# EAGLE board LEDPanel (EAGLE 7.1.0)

Size 152.65 x 130.18 mm. Coordinates in mm from the lower left corner, seen from the top.
Outline: 993 segments
Copper layers (1*16): Top 0.035mm / dielectric 1.5mm / Bottom 0.035mm
Design rules "default": minimum track width 10mil, minimum drill 24mil, track to track 8mil, track to pad 8mil, pad to pad 8mil, via to via 8mil, smd to smd 8mil, copper to edge 40mil, drill to drill 8mil, minimum pad ring 10mil, minimum via ring 8mil, stop-mask expansion 4mil, vias tented up to drill 0mil, thermal gap 10mil

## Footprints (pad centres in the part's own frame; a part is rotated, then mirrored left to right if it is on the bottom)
LED5MM = drill 0.813 octagon: A -1.27,0; K 1.27,0
SO14 = smd 0.6 x 2.2: 1 -3.81,-2.6; 2 -2.54,-2.6; 3 -1.27,-2.6; 4 0,-2.6; 5 1.27,-2.6; 6 2.54,-2.6; 7 3.81,-2.6; 8 3.81,2.6; 9 2.54,2.6; 10 1.27,2.6; 11 0,2.6; 12 -1.27,2.6; 13 -2.54,2.6; 14 -3.81,2.6
SA56-11 = drill 0.8 long: 1 -5.08,-7.62; 2 -2.54,-7.62; 3 0,-7.62; 4 2.54,-7.62; 5 5.08,-7.62; 6 5.08,7.62; 7 2.54,7.62; 8 0,7.62; 9 -2.54,7.62; 10 -5.08,7.62

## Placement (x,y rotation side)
E$1  [LED5MM]  124.84,73.03 90 top
E$2  [LED5MM]  132.46,73.03 90 top
E$3  [LED5MM]  109.6,73.03 90 top
E$4  [LED5MM]  117.22,73.03 90 top
E$5  [LED5MM]  94.36,73.03 90 top
E$6  [LED5MM]  101.98,73.03 90 top
E$7  [LED5MM]  79.12,73.03 90 top
E$8  [LED5MM]  86.74,73.03 90 top
E$9  [LED5MM]  63.88,73.03 90 top
E$10  [LED5MM]  71.5,73.03 90 top
E$11  [LED5MM]  48.64,73.03 90 top
E$12  [LED5MM]  56.26,73.03 90 top
E$13  [LED5MM]  33.4,73.03 90 top
E$14  [LED5MM]  41.02,73.03 90 top
E$15  [LED5MM]  18.16,73.03 90 top
E$16  [LED5MM]  25.78,73.03 90 top
E$17  [LED5MM]  124.84,80.64 90 top
E$18  [LED5MM]  132.46,80.64 90 top
E$19  [LED5MM]  109.6,80.64 90 top
E$20  [LED5MM]  117.22,80.64 90 top
E$21  [LED5MM]  94.36,80.64 90 top
E$22  [LED5MM]  101.98,80.64 90 top
E$23  [LED5MM]  79.12,80.64 90 top
E$24  [LED5MM]  86.74,80.64 90 top
E$25  [LED5MM]  63.88,80.64 90 top
E$26  [LED5MM]  71.5,80.64 90 top
E$27  [LED5MM]  48.64,80.64 90 top
E$28  [LED5MM]  56.26,80.64 90 top
E$29  [LED5MM]  33.4,80.64 90 top
E$30  [LED5MM]  41.02,80.64 90 top
E$31  [LED5MM]  18.16,80.64 90 top
E$32  [LED5MM]  25.78,80.64 90 top
E$33  [LED5MM]  124.84,88.27 90 top
E$34  [LED5MM]  132.46,88.27 90 top
E$35  [LED5MM]  109.6,88.27 90 top
E$36  [LED5MM]  117.22,88.27 90 top
E$37  [LED5MM]  94.36,88.27 90 top
E$38  [LED5MM]  101.98,88.27 90 top
E$39  [LED5MM]  79.12,88.27 90 top
E$40  [LED5MM]  86.74,88.27 90 top
E$41  [LED5MM]  63.88,88.27 90 top
E$42  [LED5MM]  71.5,88.27 90 top
E$43  [LED5MM]  48.64,88.27 90 top
E$44  [LED5MM]  56.26,88.27 90 top
E$45  [LED5MM]  33.4,88.27 90 top
E$46  [LED5MM]  41.02,88.27 90 top
E$47  [LED5MM]  18.16,88.27 90 top
E$48  [LED5MM]  25.78,88.27 90 top
E$49  [LED5MM]  124.84,95.89 90 top
E$50  [LED5MM]  132.46,95.89 90 top
E$51  [LED5MM]  109.6,95.89 90 top
E$52  [LED5MM]  117.22,95.89 90 top
E$53  [LED5MM]  94.36,95.89 90 top
E$54  [LED5MM]  101.98,95.89 90 top
E$55  [LED5MM]  79.12,95.89 90 top
E$56  [LED5MM]  86.74,95.89 90 top
E$57  [LED5MM]  63.88,95.89 90 top
E$58  [LED5MM]  71.5,95.89 90 top
E$59  [LED5MM]  48.64,95.89 90 top
E$60  [LED5MM]  56.26,95.89 90 top
E$61  [LED5MM]  33.4,95.89 90 top
E$62  [LED5MM]  41.02,95.89 90 top
E$63  [LED5MM]  18.16,95.89 90 top
E$64  [LED5MM]  25.78,95.89 90 top
E$65  [LED5MM]  124.84,103.5 90 top
E$66  [LED5MM]  132.46,103.5 90 top
E$67  [LED5MM]  109.6,103.5 90 top
E$68  [LED5MM]  117.22,103.5 90 top
E$69  [LED5MM]  94.36,103.5 90 top
E$70  [LED5MM]  101.98,103.5 90 top
E$71  [LED5MM]  79.12,103.5 90 top
E$72  [LED5MM]  86.74,103.5 90 top
E$73  [LED5MM]  63.88,103.5 90 top
E$74  [LED5MM]  71.5,103.5 90 top
E$75  [LED5MM]  48.64,103.5 90 top
E$76  [LED5MM]  56.26,103.5 90 top
E$77  [LED5MM]  33.4,103.5 90 top
E$78  [LED5MM]  41.02,103.5 90 top
E$79  [LED5MM]  18.16,103.5 90 top
E$80  [LED5MM]  25.78,103.5 90 top
E$81  [LED5MM]  124.84,111.12 90 top
E$82  [LED5MM]  132.46,111.12 90 top
E$83  [LED5MM]  109.6,111.12 90 top
E$84  [LED5MM]  117.22,111.12 90 top
E$85  [LED5MM]  94.36,111.12 90 top
E$86  [LED5MM]  101.98,111.12 90 top
E$87  [LED5MM]  79.12,111.12 90 top
E$88  [LED5MM]  86.74,111.12 90 top
E$89  [LED5MM]  63.88,111.12 90 top
E$90  [LED5MM]  71.5,111.12 90 top
E$91  [LED5MM]  48.64,111.12 90 top
E$92  [LED5MM]  56.26,111.12 90 top
E$93  [LED5MM]  33.4,111.12 90 top
E$94  [LED5MM]  41.02,111.12 90 top
E$95  [LED5MM]  18.16,111.12 90 top
E$96  [LED5MM]  25.78,111.12 90 top
E$97  [LED5MM]  124.84,118.75 90 top
E$98  [LED5MM]  132.46,118.75 90 top
E$99  [LED5MM]  109.6,118.75 90 top
E$100  [LED5MM]  117.22,118.75 90 top
E$101  [LED5MM]  94.36,118.75 90 top
E$102  [LED5MM]  101.98,118.75 90 top
E$103  [LED5MM]  79.12,118.75 90 top
E$104  [LED5MM]  86.74,118.75 90 top
E$105  [LED5MM]  63.88,118.75 90 top
E$106  [LED5MM]  71.5,118.75 90 top
E$107  [LED5MM]  48.64,118.75 90 top
E$108  [LED5MM]  56.26,118.75 90 top
E$109  [LED5MM]  33.4,118.75 90 top
E$110  [LED5MM]  41.02,118.75 90 top
E$111  [LED5MM]  18.16,118.75 90 top
E$112  [LED5MM]  25.78,118.75 90 top
E$113  [LED5MM]  124.84,126.36 90 top
E$114  [LED5MM]  132.46,126.36 90 top
E$115  [LED5MM]  109.6,126.36 90 top
E$116  [LED5MM]  117.22,126.36 90 top
E$117  [LED5MM]  94.36,126.36 90 top
E$118  [LED5MM]  101.98,126.36 90 top
E$119  [LED5MM]  79.12,126.36 90 top
E$120  [LED5MM]  86.74,126.36 90 top
E$121  [LED5MM]  63.88,126.36 90 top
E$122  [LED5MM]  71.5,126.36 90 top
E$123  [LED5MM]  48.64,126.36 90 top
E$124  [LED5MM]  56.26,126.36 90 top
E$125  [LED5MM]  33.4,126.36 90 top
E$126  [LED5MM]  41.02,126.36 90 top
E$127  [LED5MM]  18.16,126.36 90 top
E$128  [LED5MM]  25.78,126.36 90 top
E$139  [SO14]  142.94,99.71 180 top
E$140  [SO14]  7.81,103.49 0 top
E$141  [SO14]  138.24,53.74 180 top
E$142  [SA56-11]  81.85,53.8 0 top
E$143  [SA56-11]  95.31,53.8 0 top
E$144  [SA56-11]  108.77,53.8 0 top
E$145  [SA56-11]  122.23,53.8 0 top
E$146  [SO14]  12.26,53.83 0 top
E$147  [SA56-11]  68.65,53.77 180 top
E$148  [SA56-11]  55.19,53.77 180 top
E$149  [SA56-11]  41.72,53.77 180 top
E$150  [SA56-11]  28.26,53.77 180 top
E$151  [SO14]  138.24,23.13 180 top
E$152  [SA56-11]  81.85,23.19 0 top
E$153  [SA56-11]  95.31,23.19 0 top
E$154  [SA56-11]  108.77,23.19 0 top
E$155  [SA56-11]  122.23,23.19 0 top
E$156  [SO14]  12.26,23.22 0 top
E$157  [SA56-11]  68.65,23.16 180 top
E$158  [SA56-11]  55.19,23.16 180 top
E$159  [SA56-11]  41.72,23.16 180 top
E$160  [SA56-11]  28.26,23.16 180 top

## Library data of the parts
E$1-E$128 = led
E$139-E$141 E$146 E$151 E$156 = analog-devices
E$142-E$145 E$147-E$150 E$152-E$155 E$157-E$160 = display-kingbright

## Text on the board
Unrouted: Vcc | Q7 | Q6 | Q5 | Q4 | MR | cp | gnd | Q3 | Q2 | Q1 | Q0 | B | A | 74HC164 | A | B | Q0 | Q1 | Q2 | Q3 | gnd | 74HC164 | cp | MR | Q4 | Q5 | Q6 | Q7 | Vcc | Q7 | Q6 | Q5 | Q4 | cp | gnd | Q3 | Q2 | Q1 | Q0 | B | A | Vcc | MR | 74HC164 | 74HC164 | A | B | cp | MR | Q4 | Q5 | Q6 | Q7 | Vcc | Q0 | Q1 | Q2 | Q3 | gnd | gnd | Q3 | Q2 | Q1 | Q0 | Vcc | Q7 | Q6 | Q5 | Q4 | MR | cp | B | A | 74HC164 | 74HC164 | MR | Vcc | A | B | Q0 | Q1 | Q2 | Q3 | gnd | cp | Q4 | Q5 | Q6 | Q7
